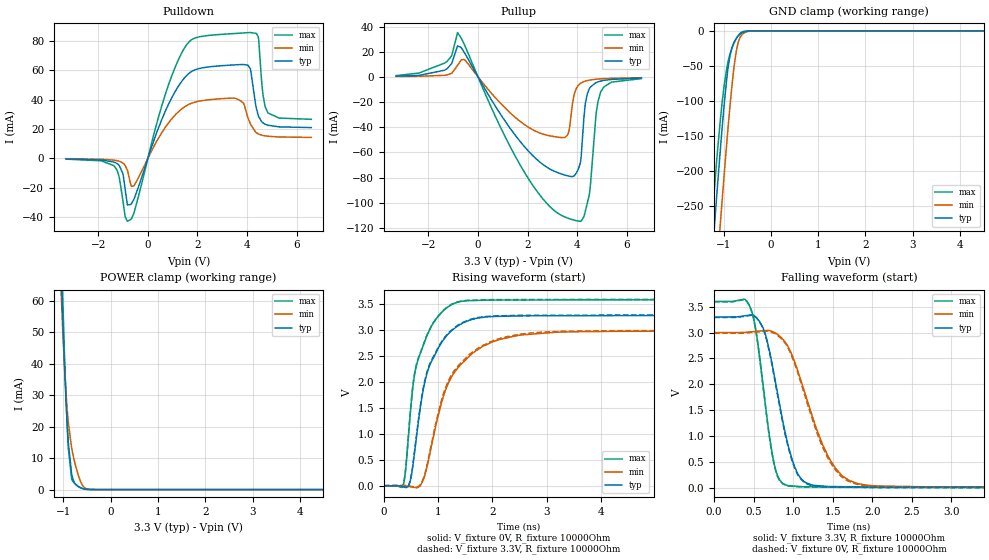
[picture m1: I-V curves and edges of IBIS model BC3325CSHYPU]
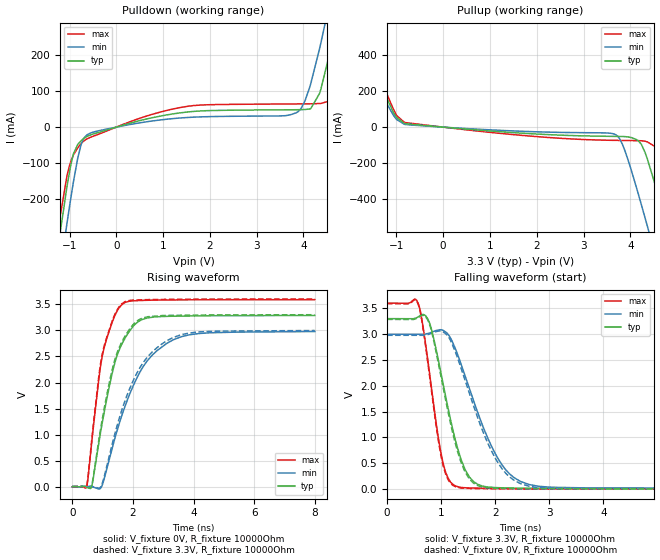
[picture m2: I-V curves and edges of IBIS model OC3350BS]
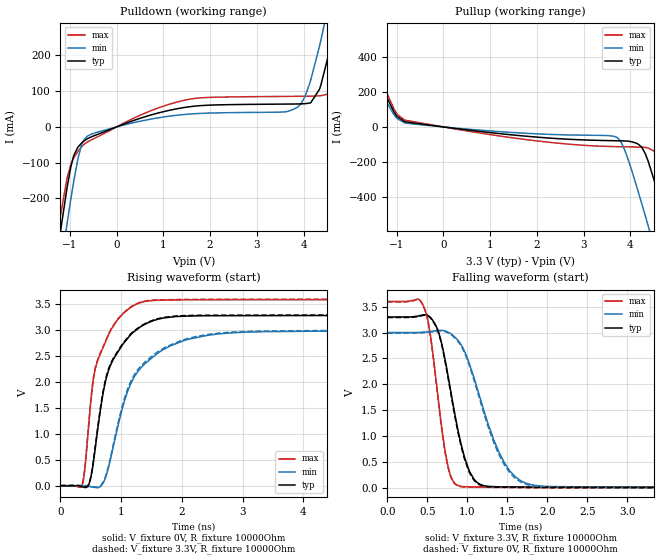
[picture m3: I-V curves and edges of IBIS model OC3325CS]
|Texas Instruments Incorporated
|Industrial Temp, Single Port 10/100Mbs Ethernet Physical Layer Transceiver
| Marketing part#   Digital Voltage Range   Package-type   #pins
|TLK105   3.3 to 3.6 V   QFN   32
|TLK106   3.3 to 3.6 V   QFN   32
[IBIS Ver]   4.0
[File name]   tlk10x.ibs
[File Rev]   1.0
[Date]   08/24/2012
[Source]   Texas Instruments Incorporated.
   Analog-eLab, HPA
   12500 TI Blvd
   Dallas, TX -75243
   For Support e-mail: elab_ibis@list.ti.com
[Notes]   Revision History:
   1.0: 08/24/2012
   - Initial version of the model
   - Initial Model generated from simulations in TISPICED
   - Model not matched to measurements
   - Models with trailing _3p3v are generated based on 3.3V
   power supply.
   - C_comp although listed in numerical order of value are
   obtained from varying PVT conditions. For PVT conditions
   for each specific value refer the buffer description under
   respective [Model]. IBIS model user is responsible for using
   appropriate C_comp to simulate for Signal Integrity.
   - Combined Pulldown/pullup non-monotonic warnings for BC3350BSHY,
   BC3350BSHYPD, BC3350BSHYPU, and OSC_TOP1 are based on
   SPICE simulations and accepted.
[Disclaimer]
  This model is designed as an aid for customers of Texas Instruments.
  TI and its licensors and suppliers make no warranties, either expressed
  or implied, with respect to this model, including the warranties of
  merchantability or fitness for a particular purpose.  The model is
  provided solely on an "as is" basis.  The entire risk as to its quality
  and performance is with the customer.
[Copyright] (C) Copyright 2012 Texas Instruments Incorporated.
   All rights reserved.
|   AFE7222 and AFE7225
[Component]   tlk10x
[Manufacturer] TI
[Package]   | 32 pin  QFN
| variable   typ   min   max
R_pkg  0.1   0.08   0.12
L_pkg  2.0nH  1.8nH  2.2nH
C_pkg  0.5pF  0.51pF  0.49pF
|-------------------------PIN------------------------------------------------
[Pin] signal_name  model_name  R_pin  L_pin C_pin
1   RXD_3/PHYAD4   BC3350BSHYPD   NA   NA   NA
2   TX_CLK   OC3350BS   NA   NA   NA
3   TXEN   BC3350BSHYPD   NA   NA   NA
4   TXD_0   BC3350BSHYPD   NA   NA   NA
5   TXD_1   IC33SHYPD   NA   NA   NA
6   TXD_2   IC33SHYPD   NA   NA   NA
7   TXD_3   BC3350BSHYPD   NA   NA   NA
8   INTB/PWDNB   BC3350BSHYPU   NA   NA   NA
9   RD-   TERM   NA   NA   NA
10   RD+   TERM   NA   NA   NA
11   TD-   TERM   NA   NA   NA
12   TD+   TERM   NA   NA   NA
13   PRBIN1   TERM   NA   NA   NA
14   AVDD33   POWER   NA   NA   NA
15   PFBOUT   TERM   NA   NA   NA
16   RBIAS   TERM   NA   NA   NA
17   LED_LINK/AN0   BC3325CSHYPU   NA   NA   NA
18   RESETB   IC33SHYPU   NA   NA   NA
19   MDIO   BC3350BSHY   NA   NA   NA
20   MDC   IC33SHY   NA   NA   NA
21   VDD33_IO   POWER   NA   NA   NA
22   XO   OSC_TOP1   NA   NA   NA
23   XI   OSC_TOP1   NA   NA   NA
24   PFBIN2   TERM   NA   NA   NA
25   RX_CLK   OC3350BS   NA   NA   NA
26   RX_DIV/MII_MODE   BC3350BSHYPD   NA   NA   NA
27   CRS/CRS_DV/LED_CFG   BC3350BSHYPU   NA   NA   NA
28   RX_ER/AMDIX_EN   BC3350BSHYPU   NA   NA   NA
29   COL/PHYAD0   BC3350BSHYPU   NA   NA   NA
30   RXD_0/PHYAD1   BC3350BSHYPD   NA   NA   NA
31   RXD_1/PHYAD2   BC3350BSHYPD   NA   NA   NA
32   RXD_2/PHYAD3   BC3350BSHYPD   NA   NA   NA
|   TERM_3p3v Model
[Model] TERM
Model_type Terminator
C_comp   1fF   1fF   1fF
| variable   typ   min   max
[Voltage Range]   3.3V   3.0V   3.6V
[POWER Clamp Reference]  3.3V   3.0V   3.6V
[GND Clamp Reference]   0.0V   0.0V   0.0V
|Operating Temperature
[Temperature Range]   25   125   -40
| Models and submodels in the file (12): BC3325CSHYPU (I/O), OC3350BS (Output), OC3325CS (Output), OSC_TOP2 (Input), OSC_TOP1 (I/O), IC33SHYPU (Input), IC33SHYPD (Input), IC33SHY (Input), BC3350BSHYPU (I/O), BC3350BSHYPD (I/O), BC3350BSHY (I/O), TERM (Terminator)
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|   Model
[Model]   BC3325CSHYPU
Model_type   I/O
Polarity   Non-Inverting
Enable   Active-Low
Vinl = 0.99
Vinh = 2.31
Vmeas = 1.65
Vref = 1.65
Cref = 1pF
Rref = 10000
|   typ   min   max
C_comp   2.034pF   1.945pF   2.081pF
[Voltage Range]   3.3   3   3.6
[Temperature Range]   25   125   -40
[Pullup Reference]   3.3   3   3.6
[Pulldown Reference]   -0   -0   -0
[Power Clamp Reference]   3.3   3   3.6
[GND Clamp Reference]   -0   -0   -0
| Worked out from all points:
|   slope of the pulldown table from 0 to 0.495 V, typ, clamps not added: 20.9 ohm
|   slope of the pullup table from 0 to 0.495 V, typ, clamps not added: 29.6 ohm
|   GND clamp passes 1 mA (typ) near -0.55 V on its own axis
|   POWER clamp passes 1 mA (typ) near -0.69 V on its own axis
|   falling waveform, V_fixture 3.3V, R_fixture 10000Ohm: 20-80 % time 264ps typ, 417ps min, 183ps max; typ from 3.3 V to 0.008 V
|   rising waveform, V_fixture 0V, R_fixture 10000Ohm: 20-80 % time 426ps typ, 627ps min, 351ps max; typ from 0.002 V to 3.29 V
|   rising waveform, V_fixture 3.3V, R_fixture 10000Ohm: 20-80 % time 423ps typ, 614ps min, 350ps max; typ from 0.008 V to 3.3 V
|   falling waveform, V_fixture 0V, R_fixture 10000Ohm: 20-80 % time 262ps typ, 411ps min, 182ps max; typ from 3.29 V to 0.002 V
[Pulldown]
|   Voltage   I(typ)   I(min)   I(max)
-3.3V     -411.3uA   -235.9uA   -545.7uA
-1.369V   -2.548mA   -1.234mA   -5.013mA
-914.1mV  -21.57mA   -4.879mA   -39.96mA
-686.4mV  -31.47mA   -18.14mA   -41.64mA
976.8mV   41.79mA    27.24mA    56.91mA
2.224V    61.83mA    39.46mA    83.37mA
3.561V    63.83mA    40.84mA    85.24mA
4.036V    63.55mA    27.69mA    85.77mA
4.382V    33.81mA    17.41mA    85.13mA
4.65V     24.1mA     15.58mA    42.69mA
4.838V    22.6mA     15.08mA    31.16mA
6.59V     20.98mA    14.27mA    26.62mA
[GND Clamp]
|   Voltage   I(typ)   I(min)   I(max)
-3.3V     -2.327A    -2.431A    -2.267A
-1.251V   -331.9mA   -441.7mA   -275.1mA
-1.142V   -233.7mA   -342.1mA   -183mA
-1.063V   -165.7mA   -271.3mA   -124mA
-993.3mV  -110.6mA   -211.3mA   -81.74mA
-933.9mV  -69.59mA   -161.9mA   -54.23mA
-864.6mV  -35.64mA   -108.2mA   -33.34mA
-795.3mV  -19.11mA   -61.58mA   -20.33mA
-735.9mV  -11.53mA   -31.53mA   -11.75mA
-676.5mV  -6.299mA   -13.89mA   -5.533mA
-597.3mV  -2.187mA   -4.675mA   -1.421mA
6.59V     0A         0A         0A
[Pullup]
|   Voltage   I(typ)   I(min)   I(max)
-3.3V     620.4uA    341.3uA    995.8uA
-1.261V   6.274mA    1.513mA    12.07mA
-825mV    24.56mA    9.145mA    35.23mA
1.531V    -47.14mA   -32.67mA   -64.1mA
3.214V    -76.12mA   -47.92mA   -108.3mA
3.63V     -78.72mA   -45.56mA   -112.3mA
3.877V    -78.75mA   -14.11mA   -113.9mA
4.125V    -68.66mA   -5.319mA   -114.8mA
4.412V    -13.25mA   -2.932mA   -100.2mA
4.769V    -4.501mA   -1.857mA   -28.77mA
4.947V    -3.328mA   -1.565mA   -12.14mA
6.59V     -948.7uA   -633.5uA   -1.387mA
[POWER Clamp]
|   Voltage   I(typ)   I(min)   I(max)
-3.3V     1.556A     1.474A     1.625A
-1.063V   77.92mA    68.87mA    89.09mA
-1.023V   59.36mA    54.46mA    67.03mA
-1.013V   55.03mA    51.11mA    61.8mA
-943.8mV  28.62mA    31.12mA    29.69mA
-894.3mV  14.97mA    21.34mA    13.29mA
-825mV    5.162mA    13.39mA    3.578mA
-755.7mV  1.97mA     8.538mA    1.911mA
-636.9mV  582.3uA    2.669mA    625.9uA
-547.8mV  178.6uA    599.2uA    152.1uA
-409.2mV  20.75uA    41.14uA    21.99uA
6.59V     0A         0A         0A
[Ramp]
R_load = 10000
|   typ   min   max
dV/dt_r   1.97317/4.23784e-10   1.79086/6.21111e-10   2.15424/3.50065e-10
dV/dt_f   1.97506/2.63195e-10   1.79287/4.17282e-10   2.15581/1.83027e-10
[Falling Waveform]
V_fixture = 3.3V
V_fixture_min = 3V
V_fixture_max = 3.6V
R_fixture = 10000Ohm
C_fixture = 0F
|   Time   V(typ)   V(min)   V(max)
0s        3.3V       2.999V     3.6V
467.3ps   3.341V     3.014V     3.45V
545.3ps   3.271V     3.024V     2.884V
633.2ps   3.038V     3.036V     1.815V
751.9ps   2.251V     3.012V     530.5mV
918.7ps   943.6mV    2.773V     51.29mV
1.148ns   113.3mV    1.836V     23.9mV
1.468ns   27.39mV    544.1mV    19.57mV
1.816ns   21.11mV    85.43mV    14.86mV
8ns       8.116mV    10.82mV    6.983mV
[Rising Waveform]
V_fixture = 0V
V_fixture_min = 0V
V_fixture_max = 0V
R_fixture = 10000Ohm
C_fixture = 0F
|   Time   V(typ)   V(min)   V(max)
0s        1.877mV    2.333mV    1.938mV
358ps     -15.61mV   3.395mV    25.05mV
491.7ps   128.5mV    -13.59mV   1.467V
564.3ps   639.9mV    -26.25mV   2.144V
678.4ps   1.56V      18.46mV    2.574V
856.2ps   2.355V     670.4mV    3.034V
1.251ns   2.994V     2.111V     3.495V
1.816ns   3.247V     2.686V     3.577V
2.507ns   3.278V     2.908V     3.583V
8ns       3.29V      2.987V     3.592V
[Rising Waveform]
V_fixture = 3.3V
V_fixture_min = 3V
V_fixture_max = 3.6V
R_fixture = 10000Ohm
C_fixture = 0F
|   Time   V(typ)   V(min)   V(max)
0s        8.115mV    10.82mV    6.983mV
358ps     -8.81mV    11.83mV    32.89mV
491.7ps   142.1mV    -3.915mV   1.493V
564.3ps   671.9mV    -15.65mV   2.167V
661.4ps   1.47V      9.278mV    2.541V
842.7ps   2.346V     641.7mV    3.016V
1.251ns   3.007V     2.151V     3.504V
1.775ns   3.252V     2.684V     3.584V
2.681ns   3.288V     2.945V     3.591V
8ns       3.3V       2.999V     3.6V
[Falling Waveform]
|Gnd
V_fixture = 0V
V_fixture_min = 0V
V_fixture_max = 0V
R_fixture = 10000Ohm
C_fixture = 0F
|   Time   V(typ)   V(min)   V(max)
0s        3.29V      2.987V     3.592V
467.3ps   3.331V     3.001V     3.439V
545.3ps   3.264V     3.011V     2.864V
633.2ps   3.021V     3.023V     1.79V
751.9ps   2.215V     2.992V     508.1mV
918.7ps   902.8mV    2.75V      43.82mV
1.083ns   196.2mV    2.109V     22.09mV
1.435ns   21.33mV    591mV      14.69mV
1.804ns   14.99mV    72.3mV     10.08mV
8ns       1.878mV    2.335mV    1.939mV
|   Model
[Model]   OC3350BS
Model_type   Output
Polarity   Non-Inverting
Vmeas = 1.65
Vref = 1.65
Cref = 1pF
Rref = 10000
|   typ   min   max
C_comp   1.804pF   1.746pF   1.890pF
[Voltage Range]   3.3   3   3.6
[Temperature Range]   25   125   -40
[Pullup Reference]   3.3   3   3.6
[Pulldown Reference]   -0   -0   -0
[Power Clamp Reference]   3.3   3   3.6
[GND Clamp Reference]   -0   -0   -0
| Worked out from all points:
|   slope of the pulldown table from 0 to 0.495 V, typ, clamps not added: 27.8 ohm
|   slope of the pullup table from 0 to 0.495 V, typ, clamps not added: 45 ohm
|   falling waveform, V_fixture 3.3V, R_fixture 10000Ohm: 20-80 % time 421ps typ, 668ps min, 289ps max; typ from 3.3 V to 0.008 V
|   rising waveform, V_fixture 0V, R_fixture 10000Ohm: 20-80 % time 726ps typ, 1.18ns min, 536ps max; typ from 0 V to 3.29 V
|   rising waveform, V_fixture 3.3V, R_fixture 10000Ohm: 20-80 % time 710ps typ, 1.13ns min, 533ps max; typ from 0.008 V to 3.3 V
|   falling waveform, V_fixture 0V, R_fixture 10000Ohm: 20-80 % time 413ps typ, 647ps min, 286ps max; typ from 3.29 V to 0 V
[Pulldown]
|   Voltage   I(typ)   I(min)   I(max)
-3.3V     -2.327A    -2.431A    -2.267A
-1.29V    -370.6mA   -479.5mA   -315.1mA
-1.053V   -163.3mA   -264.6mA   -133.8mA
-755.7mV  -37.94mA   -49.73mA   -45.97mA
-547.8mV  -21.41mA   -16.07mA   -27.9mA
1.531V    41.99mA    26.76mA    57.74mA
3.848V    48.11mA    39.9mA     64.18mA
4.155V    51.04mA    119.8mA    64.49mA
4.531V    188.7mA    327.6mA    71.26mA
4.759V    329.5mA    469.5mA    170.8mA
5.263V    660.8mA    794.1mA    502.6mA
6.59V     1.555A     1.666A     1.42A
[Pullup]
|   Voltage   I(typ)   I(min)   I(max)
-3.3V     1.546A     1.464A     1.616A
-2.033V   691.9mA    634mA      738.7mA
-1.379V   264.5mA    224.9mA    296.6mA
-1.063V   81.82mA    65.26mA    98.47mA
-825mV    19.84mA    15.21mA    25.77mA
3.67V     -51.33mA   -39.85mA   -73.29mA
3.897V    -52.85mA   -140.6mA   -74.13mA
4.165V    -74.43mA   -365.8mA   -75.02mA
4.363V    -175.9mA   -548mA     -81.64mA
4.798V    -566.5mA   -962.6mA   -243.4mA
5.293V    -1.043A    -1.443A    -692mA
6.59V     -2.317A    -2.717A    -1.961A
[Ramp]
R_load = 10000
|   typ   min   max
dV/dt_r   1.97128/7.26236e-10   1.78613/1.18083e-09   2.15306/5.3647e-10
dV/dt_f   1.97487/4.21057e-10   1.79079/6.67275e-10   2.15599/2.89325e-10
[Falling Waveform]
V_fixture = 3.3V
V_fixture_min = 3V
V_fixture_max = 3.6V
R_fixture = 10000Ohm
C_fixture = 0F
|   Time   V(typ)   V(min)   V(max)
0s        3.3V       2.997V     3.6V
576.4ps   3.336V     2.997V     3.596V
783.4ps   3.224V     3.02V      2.266V
989.2ps   2.289V     3.085V     743.1mV
1.13ns    1.566V     2.995V     210.4mV
1.267ns   939.4mV    2.709V     61.6mV
1.604ns   142.9mV    1.702V     21.14mV
2.059ns   28.58mV    581.5mV    13.83mV
2.466ns   19.49mV    150mV      10.85mV
8ns       8.337mV    12.33mV    6.674mV
[Rising Waveform]
V_fixture = 0V
V_fixture_min = 0V
V_fixture_max = 0V
R_fixture = 10000Ohm
C_fixture = 0F
|   Time   V(typ)   V(min)   V(max)
0s        38.66uV    676.4uV    381nV
459.3ps   -3.666mV   1.659mV    -17.5mV
505.8ps   -13.54mV   1.759mV    104.1mV
625.8ps   -12.55mV   2.016mV    766.2mV
989.2ps   1.229V     37.93mV    2.508V
1.366ns   2.297V     847mV      3.23V
1.622ns   2.721V     1.346V     3.487V
2.341ns   3.215V     2.307V     3.574V
3.337ns   3.271V     2.82V      3.583V
8ns       3.285V     2.978V     3.588V
[Rising Waveform]
V_fixture = 3.3V
V_fixture_min = 3V
V_fixture_max = 3.6V
R_fixture = 10000Ohm
C_fixture = 0F
|   Time   V(typ)   V(min)   V(max)
0s        8.337mV    12.33mV    6.674mV
472.8ps   1.486mV    13.2mV     7.034mV
625.8ps   1.948mV    13.48mV    803.9mV
878ps     904.3mV    -25.44mV   2.128V
989.2ps   1.297V     68.99mV    2.544V
1.366ns   2.361V     932.4mV    3.254V
1.622ns   2.763V     1.449V     3.505V
2.341ns   3.24V      2.384V     3.587V
3.337ns   3.288V     2.865V     3.595V
8ns       3.3V       2.997V     3.6V
[Falling Waveform]
|Gnd
V_fixture = 0V
V_fixture_min = 0V
V_fixture_max = 0V
R_fixture = 10000Ohm
C_fixture = 0F
|   Time   V(typ)   V(min)   V(max)
0s        3.285V     2.978V     3.588V
576.4ps   3.324V     2.978V     3.579V
769.6ps   3.234V     2.996V     2.325V
989.2ps   2.227V     3.059V     692.6mV
1.13ns    1.493V     2.957V     182.9mV
1.267ns   871.9mV    2.647V     46.23mV
1.604ns   113.1mV    1.603V     12.41mV
2.025ns   15.9mV     557.7mV    6.699mV
2.466ns   8.745mV    108mV      3.822mV
8ns       38.64uV    676.6uV    381.1nV
|   Model
[Model]   OC3325CS
Model_type   Output
Polarity   Non-Inverting
Vmeas = 1.65
Vref = 1.65
Cref = 1pF
Rref = 10000
|   typ   min   max
C_comp   1.918pF   1.832pF   1.981pF
[Voltage Range]   3.3   3   3.6
[Temperature Range]   25   125   -40
[Pullup Reference]   3.3   3   3.6
[Pulldown Reference]   -0   -0   -0
[Power Clamp Reference]   3.3   3   3.6
[GND Clamp Reference]   -0   -0   -0
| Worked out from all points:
|   slope of the pulldown table from 0 to 0.495 V, typ, clamps not added: 20.9 ohm
|   slope of the pullup table from 0 to 0.495 V, typ, clamps not added: 29.6 ohm
|   falling waveform, V_fixture 3.3V, R_fixture 10000Ohm: 20-80 % time 252ps typ, 398ps min, 176ps max; typ from 3.3 V to 0.006 V
|   rising waveform, V_fixture 0V, R_fixture 10000Ohm: 20-80 % time 408ps typ, 586ps min, 345ps max; typ from 0 V to 3.29 V
|   rising waveform, V_fixture 3.3V, R_fixture 10000Ohm: 20-80 % time 405ps typ, 569ps min, 344ps max; typ from 0.006 V to 3.3 V
|   falling waveform, V_fixture 0V, R_fixture 10000Ohm: 20-80 % time 250ps typ, 391ps min, 175ps max; typ from 3.29 V to 0 V
[Pulldown]
|   Voltage   I(typ)   I(min)   I(max)
-3.3V     -2.327A    -2.431A    -2.267A
-1.28V    -362.3mA   -470.7mA   -308.4mA
-1.063V   -173.2mA   -273.9mA   -145.8mA
-825mV    -56.23mA   -88.49mA   -68.11mA
-617.1mV  -32.56mA   -25.41mA   -41.69mA
1.422V    53.77mA    34.45mA    73.75mA
3.67V     63.93mA    43.7mA     85.36mA
4.155V    67.49mA    131.1mA    85.95mA
4.541V    204.2mA    343.2mA    92.38mA
4.719V    313.6mA    454.2mA    158.8mA
5.234V    651.6mA    785.8mA    492.6mA
6.59V     1.57A      1.681A     1.435A
[Pullup]
|   Voltage   I(typ)   I(min)   I(max)
-3.3V     1.556A     1.474A     1.626A
-1.983V   665mA      609mA      711.7mA
-1.241V   184.7mA    152.9mA    212.7mA
-825mV    29.69mA    22.51mA    38.77mA
3.66V     -78.89mA   -54.56mA   -112.6mA
3.907V    -80.65mA   -152.5mA   -114mA
4.244V    -115.9mA   -439.3mA   -115.8mA
4.382V    -197.7mA   -567.6mA   -120.6mA
4.6V      -384.1mA   -773.5mA   -154.2mA
4.818V    -586.7mA   -982.3mA   -268.2mA
5.273V    -1.024A    -1.424A    -675mA
6.59V     -2.318A    -2.718A    -1.962A
[Ramp]
R_load = 10000
|   typ   min   max
dV/dt_r   1.97432/4.06248e-10   1.79238/5.8305e-10   2.15541/3.4353e-10
dV/dt_f   1.97622/2.52167e-10   1.7944/3.97933e-10   2.15697/1.76184e-10
[Falling Waveform]
V_fixture = 3.3V
V_fixture_min = 3V
V_fixture_max = 3.6V
R_fixture = 10000Ohm
C_fixture = 0F
|   Time   V(typ)   V(min)   V(max)
0s        3.3V       2.999V     3.6V
461.3ps   3.343V     3.01V      3.478V
535.4ps   3.297V     3.019V     2.981V
625.9ps   3.069V     3.039V     1.857V
747.8ps   2.259V     3.015V     491.4mV
904.6ps   962.4mV    2.805V     33.92mV
1.12ns    107.7mV    1.944V     16.21mV
1.464ns   18.5mV     483.1mV    13.12mV
1.799ns   14.63mV    61.05mV    10.13mV
8ns       6.246mV    8.705mV    5.043mV
[Rising Waveform]
V_fixture = 0V
V_fixture_min = 0V
V_fixture_max = 0V
R_fixture = 10000Ohm
C_fixture = 0F
|   Time   V(typ)   V(min)   V(max)
0s        9.473uV    226.5uV    -60.75nV
352.2ps   -16.15mV   1.381mV    -221.9uV
493.7ps   130.9mV    -16.25mV   1.549V
578ps     773.5mV    -31.46mV   2.281V
682.3ps   1.649V     17.65mV    2.616V
852.2ps   2.398V     665.3mV    3.048V
1.106ns   2.843V     1.824V     3.397V
1.333ns   3.077V     2.288V     3.54V
2.59ns    3.28V      2.928V     3.588V
8ns       3.291V     2.988V     3.592V
[Rising Waveform]
V_fixture = 3.3V
V_fixture_min = 3V
V_fixture_max = 3.6V
R_fixture = 10000Ohm
C_fixture = 0F
|   Time   V(typ)   V(min)   V(max)
0s        6.245mV    8.706mV    5.043mV
352.2ps   -9.399mV   9.816mV    6.99mV
493.7ps   144.8mV    -6.523mV   1.576V
556.7ps   609.6mV    -17.06mV   2.183V
665.1ps   1.557V     7.497mV    2.583V
852.2ps   2.421V     700.4mV    3.058V
1.106ns   2.859V     1.871V     3.405V
1.333ns   3.09V      2.322V     3.548V
2.59ns    3.29V      2.943V     3.596V
8ns       3.3V       2.999V     3.6V
[Falling Waveform]
|Gnd
V_fixture = 0V
V_fixture_min = 0V
V_fixture_max = 0V
R_fixture = 10000Ohm
C_fixture = 0F
|   Time   V(typ)   V(min)   V(max)
0s        3.291V     2.988V     3.592V
461.3ps   3.333V     2.998V     3.468V
535.4ps   3.286V     3.008V     2.963V
625.9ps   3.053V     3.026V     1.833V
747.8ps   2.225V     3.001V     469.5mV
887.4ps   1.044V     2.82V      33.83mV
1.12ns    92.08mV    1.895V     10.97mV
1.464ns   10.84mV    440.5mV    7.732mV
1.799ns   7.635mV    43.88mV    4.589mV
8ns       9.474uV    225.9uV    -60.75nV
